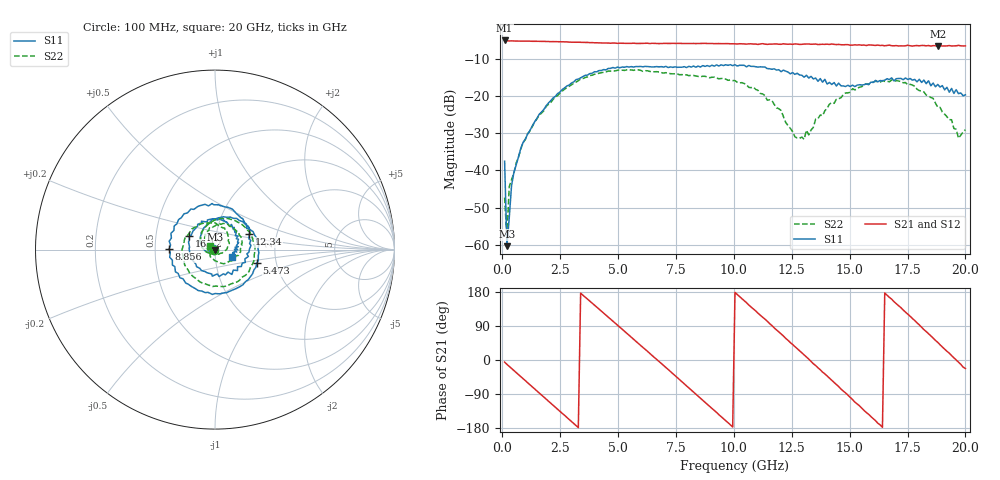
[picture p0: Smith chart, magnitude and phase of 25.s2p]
!Agilent Technologies,N5230C,MY49001569,A.09.33.09
!Agilent N5230C: A.09.33.09
!Date: Monday, July 27, 2015 17:32:06
!Correction: S11(Full 2 Port(1,2))
!S21(Full 2 Port(1,2))
!S12(Full 2 Port(1,2))
!S22(Full 2 Port(1,2))
!S2P File: Measurements: S11, S21, S12, S22:
# Hz S  dB  R 50
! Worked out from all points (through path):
!   201 points, 100 MHz to 20 GHz, reference 50 ohm
!   highest |S21| = -5.07 dB at 100 MHz (marker M1); lowest = -6.7 dB at 18.81 GHz (marker M2)
!   group delay of S21, straight-line fit = 153 ps
!   lowest |S11| = -60.4 dB at 199.5 MHz (marker M3), VSWR 1.00, Z = 49.9 + j0.0116 ohm
!   |S11| at or under -10 dB: start of sweep to end of sweep
!   |S22| runs from -58.0 to -12.9 dB; largest |S21 - S12| = 0.016
!   S11 on the Smith chart (normalised r, x): 100 MHz: 0.98, +0.01; 5.473 GHz: 1.58, -0.26; 8.856 GHz: 0.59, +0.00; 12.34 GHz: 1.44, +0.26; 16.12 GHz: 0.74, +0.12; 20 GHz: 1.21, -0.10
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1e8  -37.52 153.5  -5.07 -5.6  -5.09 -5.9  -47.29 -157.5
1.995e8  -60.36 173.0  -5.16 -11.4  -5.18 -11.2  -58.00 -6.7
2.99e8  -52.87 -74.1  -5.21 -16.9  -5.15 -16.8  -44.39 -50.0
4.98e8  -40.66 -88.7  -5.22 -27.6  -5.23 -27.3  -40.79 -87.8
8.96e8  -32.50 -130.8  -5.24 -49.1  -5.23 -49.0  -32.54 -126.9
1.9905e9  -21.90 161.3  -5.35 -108.4  -5.35 -108.4  -22.26 164.6
3.483e9  -14.79 80.0  -5.63 170.9  -5.60 171.2  -15.31 83.1
5.473e9  -12.22 -18.2  -5.85 65.3  -5.83 65.4  -12.94 -17.1
6.7665e9  -12.18 -80.4  -5.91 -3.7  -5.87 -3.9  -13.54 -78.5
7.9605e9  -12.35 -137.6  -5.89 -68.5  -5.85 -68.3  -14.33 -137.5
8.856e9  -11.83 179.2  -5.89 -117.1  -5.85 -117.2  -14.90 175.3
1.005e10  -11.60 120.7  -5.98 178.2  -5.96 177.9  -15.87 111.7
1.1244e10  -12.19 67.7  -5.93 112.9  -5.94 112.8  -19.45 47.7
1.23385e10  -13.56 24.6  -6.08 52.1  -6.00 52.5  -27.96 -29.1
1.3433e10  -15.41 -26.4  -6.07 -9.9  -6.02 -8.4  -28.44 -176.3
1.4826e10  -17.45 -114.1  -6.20 -86.8  -6.18 -87.4  -19.17 114.9
1.61195e10  -15.81 152.2  -6.41 -160.2  -6.46 -160.0  -16.05 63.5
1.67165e10  -15.58 115.3  -6.33 165.3  -6.50 165.6  -16.18 38.5
1.79105e10  -16.21 58.1  -6.43 98.1  -6.46 98.4  -18.17 -16.4
1.8806e10  -16.89 23.9  -6.65 46.5  -6.44 46.6  -23.03 -75.9
1.97015e10  -19.38 -5.2  -6.39 -5.8  -6.62 -5.9  -31.35 -174.2
2e10  -19.68 -23.8  -6.53 -22.5  -6.53 -22.9  -29.06 147.6
